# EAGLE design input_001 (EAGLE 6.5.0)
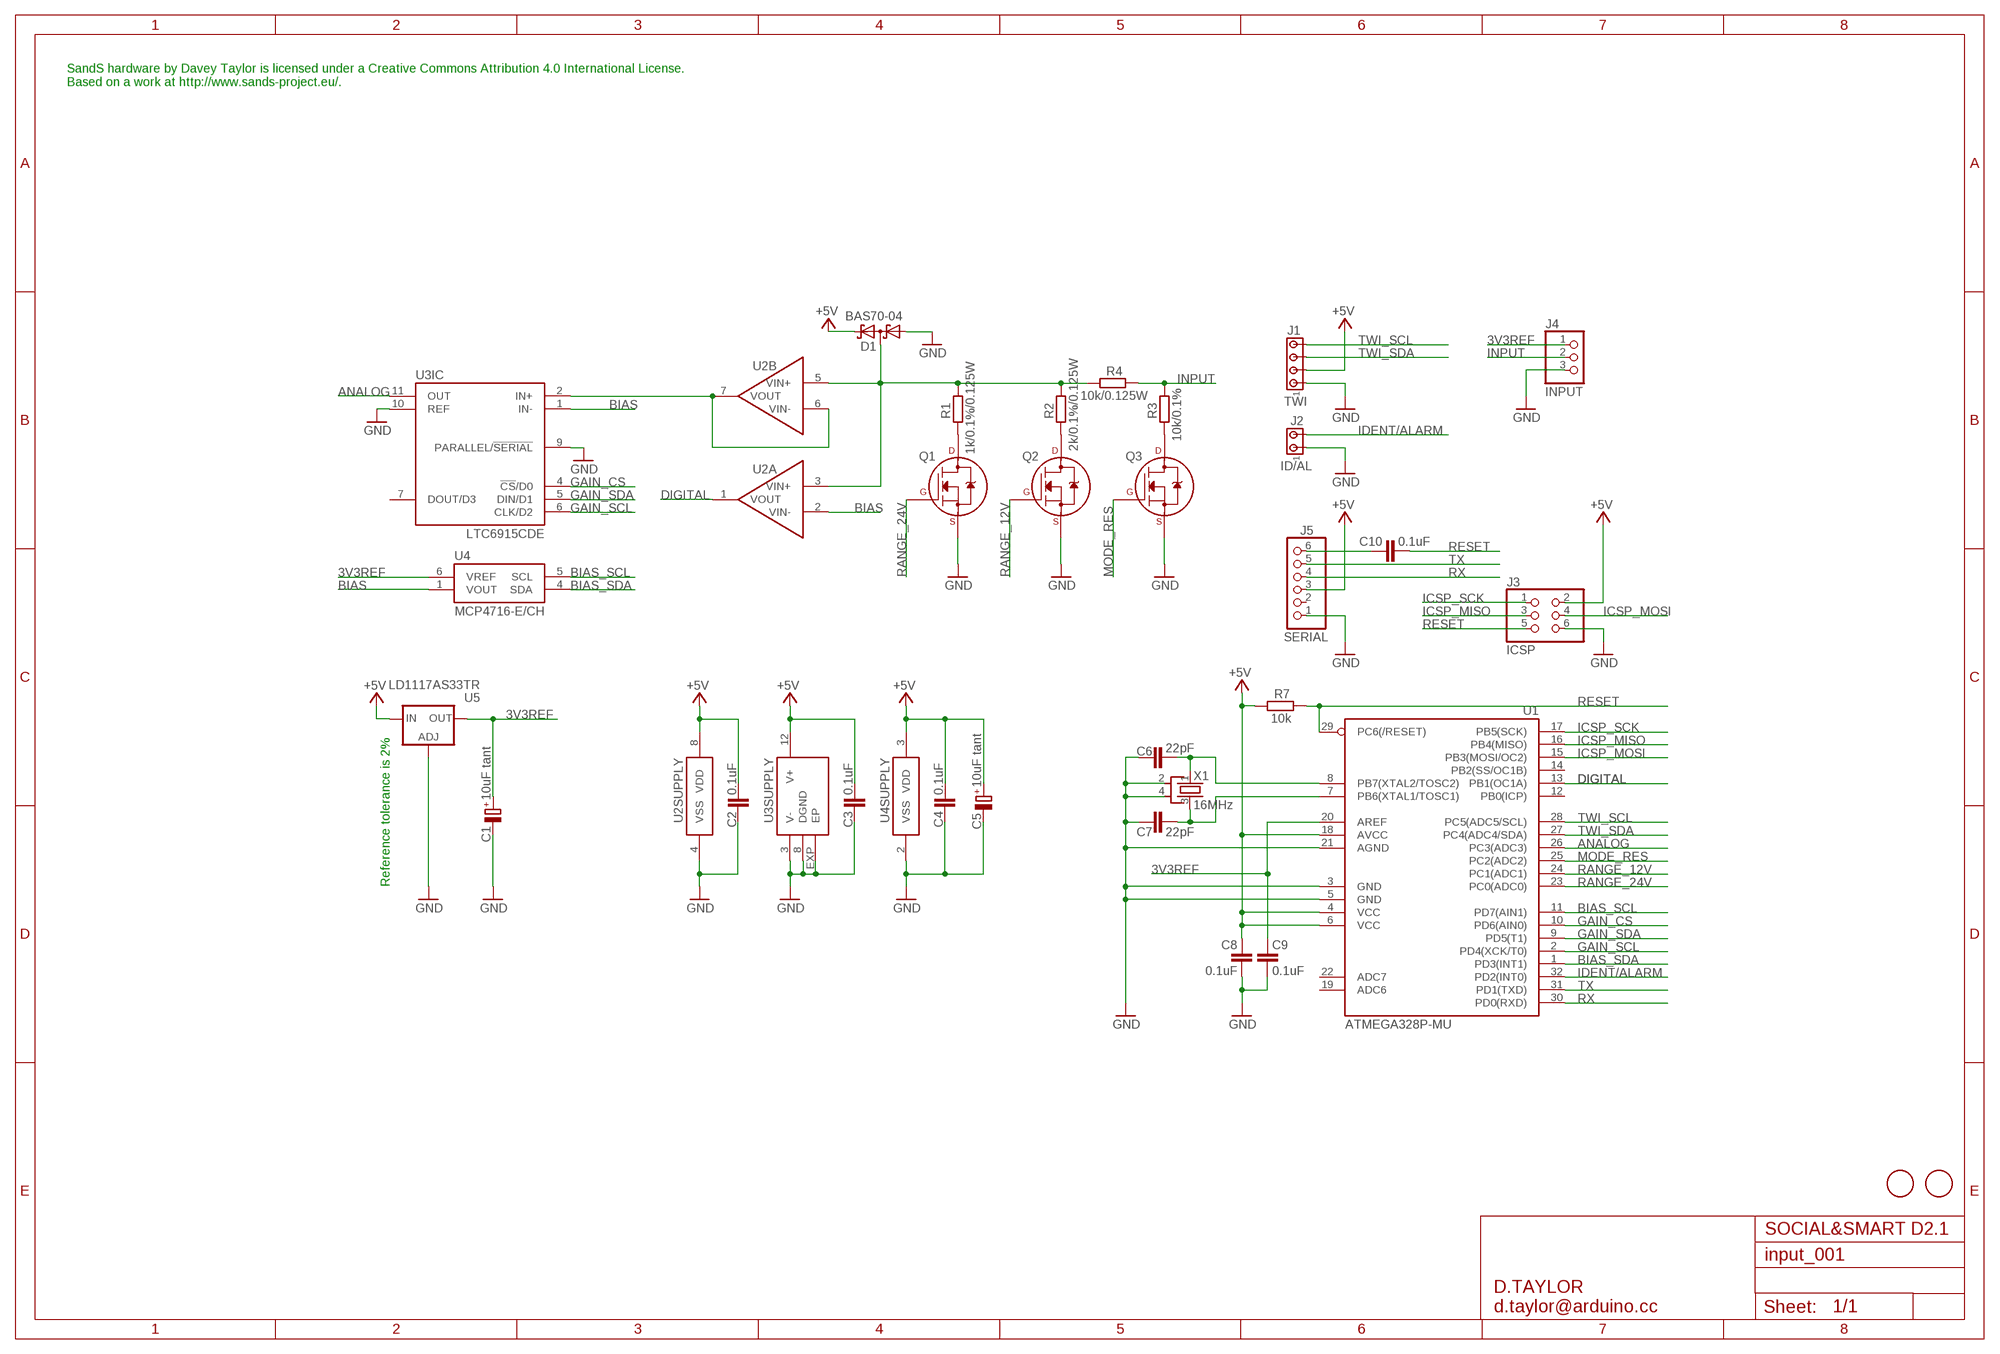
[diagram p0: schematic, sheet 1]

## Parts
C1  10uF tant  CPOL-EUSMCB  [SMC_B]
C2  0.1uF  C-EUC0603  [C0603]
C3  0.1uF  C-EUC0603  [C0603]
C4  0.1uF  C-EUC0603  [C0603]
C5  10uF tant  CPOL-EUSMCB  [SMC_B]
C6  22pF  C-EUC0603  [C0603]
C7  22pF  C-EUC0603  [C0603]
C8  0.1uF  C-EUC0603  [C0603]
C9  0.1uF  C-EUC0603  [C0603]
C10  0.1uF  C-EUC0603  [C0603]
D1  BAS70-04  [SOT23]
J1  TWI  MTA04-100  [10X04MTA]
J2  ID/AL  MTA02-100  [10X02MTA]
J3  ICSP  PINHD-2X3  [2X03]
J4  INPUT  MKDS_1,5/3-5,08  [MKDS1,5/3-5,08]
J5  SERIAL  PINHD-1X6  [1X06]
Q1  2N7002_SOT23  [SOT-23]
Q2  2N7002_SOT23  [SOT-23]
Q3  2N7002_SOT23  [SOT-23]
R1  1k/0.1%/0.125W  R-EU_R0603  [R0603]
R2  2k/0.1%/0.125W  R-EU_R0603  [R0603]
R3  10k/0.1%  R-EU_R0603  [R0603]
R4  10k/0.125W  R-EU_R0603  [R0603]
R7  10k  R-EU_R0603  [R0603]
U1  ATMEGA328P-MU  [MLF32-M1-A]
U2  MCP6402-E/SN  [SO8]
U3  LTC6915CDE  [DFN12]
U4  MCP4716-E/CH  [SOT-23-6]
U5  LD1117AS33TR  LD117AS33TR  [SOT223]
U$5  FIDUCIALMOUNT  [FIDUCIA-MOUNT]
U$6  FIDUCIALMOUNT  [FIDUCIA-MOUNT]
X1  16MHz  CRYSTAL-KX7  [XTAL-3.2-2.5]

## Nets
3V3REF: C1.+ C9.1 J4.1 U1.20(AREF) U4.6(VREF) U5.4(OUT)
+5V: C2.1 C3.1 C4.1 C5.+ C8.1 D1.2(C2) J1.2 J3.2 J5.3 R7.1 U1.4(VCC) U1.6(VCC) U1.18(AVCC) U2.8(SUPPLY:VDD) U3.12(SUPPLY:V+) U4.3(VDD) U5.3(IN)
ANALOG: U1.26(PC3(ADC3)) U3.11(IC:OUT)
BIAS: U2.2(A:VIN-) U3.1(IC:IN-) U4.1(VOUT)
BIAS_SCL: U1.11(PD7(AIN1)) U4.5(SCL)
BIAS_SDA: U1.1(PD3(INT1)) U4.4(SDA)
DIGITAL: U1.13(PB1(OC1A)) U2.1(A:VOUT)
GAIN_CS: U1.10(PD6(AIN0)) U3.4(IC:!CS!/D0)
GAIN_SCL: U1.2(PD4(XCK/T0)) U3.6(IC:CLK/D2)
GAIN_SDA: U1.9(PD5(T1)) U3.5(IC:DIN/D1)
GND: C1.- C2.2 C3.2 C4.2 C5.- C6.1 C7.1 C8.2 C9.2 D1.1(A1) J1.1 J2.1 J3.6 J4.3 J5.1 Q1.2(S) Q2.2(S) Q3.2(S) U1.3(GND) U1.5(GND) U1.21(AGND) U2.4(SUPPLY:VSS) U3.3(SUPPLY:V-) U3.8(SUPPLY:DGND) U3.9(IC:PARALLEL/!SERIAL) U3.10(IC:REF) U3.EXP(SUPPLY:EP) U4.2(VSS) U5.1(ADJ) X1.2(SH1) X1.4(SH2)
ICSP_MISO: J3.3 U1.16(PB4(MISO))
ICSP_MOSI: J3.4 U1.15(PB3(MOSI/OC2))
ICSP_SCK: J3.1 U1.17(PB5(SCK))
IDENT/ALARM: J2.2 U1.32(PD2(INT0))
INPUT: J4.2 R3.2 R4.2
MODE_RES: Q3.1(G) U1.25(PC2(ADC2))
N$1: Q1.3(D) R1.1
N$2: Q2.3(D) R2.1
N$3: Q3.3(D) R3.1
N$4: D1.3(C1A2) R1.2 R2.2 R4.1 U2.3(A:VIN+) U2.5(B:VIN+)
N$5: U2.6(B:VIN-) U2.7(B:VOUT) U3.2(IC:IN+)
N$6: C6.2 U1.8(PB7(XTAL2/TOSC2)) X1.1(X1)
N$7: C7.2 U1.7(PB6(XTAL1/TOSC1)) X1.3(X2)
N$9: C10.1 J5.6
RANGE_12V: Q2.1(G) U1.24(PC1(ADC1))
RANGE_24V: Q1.1(G) U1.23(PC0(ADC0))
RESET: C10.2 J3.5 R7.2 U1.29(PC6(/RESET))
RX: J5.4 U1.30(PD0(RXD))
TWI_SCL: J1.4 U1.28(PC5(ADC5/SCL))
TWI_SDA: J1.3 U1.27(PC4(ADC4/SDA))
TX: J5.5 U1.31(PD1(TXD))
Unconnected: J5.2 U1.12(PB0(ICP)) U1.14(PB2(SS/OC1B)) U1.19(ADC6) U1.22(ADC7) U3.7(IC:DOUT/D3)

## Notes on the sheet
- SandS hardware by Davey Taylor is licensed under a Creative Commons Attribution 4.0 International License.
  Based on a work at http://www.sands-project.eu/.
- Reference tolerance is 2%
- SOCIAL&SMART D2.1
- D.TAYLOR
  d.taylor@arduino.cc

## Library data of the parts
C1 C5 = rcl:CPOL-EU: POLARIZED CAPACITOR, European symbol
C2-C4 C6-C10 = rcl:C-EU: CAPACITOR, European symbol
D1 = diode:BAS70-04: Silicon Schottky Diodes General-purpose diode for high-speed switching
J1 = con-amp:MTA04-100: AMP connector
J2 = con-amp:MTA02-100: AMP connector
J3 = pinhead:PINHD-2X3: PIN HEADER
J4 = d_taylor:MKDS_1,5/3-5,08: MKDSN 1,5/ 3-5,08 Printklemme Nennstrom: 13,5 A Nennspannung: 250 V Rastermaß: 5,08 mm Polzahl: 3 Anschlussart: Schraubanschluss Montage: Löten Anschlussrichtung Leiter/Platine: 0 ° Artikelnummer: 1729131 Source: http://eshop.phoenixcontact.com .. 1729131.pdf; MPN: SMKDSN1,5/3-5,08; OC_FARNELL: 1792904; OC_NEWARK: 70R0299
J5 = pinhead:PINHD-1X6: PIN HEADER
Q1-Q3 = d_taylor:2N700*: 2N7000, 2N7002, NDS7002A N-channel enhancement mode MOSFET
R1-R4 R7 = rcl:R-EU_: RESISTOR, European symbol
U1 = d_taylor:ATMEGA*: MICROCONTROLLER 8 Kbytes FLASH 1 kbytes SRAM 512 bytes EEPROM USART 6-channel 10 bit ADC 2-channel 8 bit ADC Source: avr.lbr
U2 = d_taylor:MCP6402
U3 = d_taylor:LTC6915*DE
U4 = d_taylor:MCP47*6
U5 = v-reg:LD117A?*: Low drop fixed and adjustable positive voltage regulators 1 A Source: http://www.st.com/stonline/products/literature/ds/7194/ld1117axx.pdf
U$5 U$6 = SmartPrj:FIDUCIALMOUNT
X1 = d_taylor:CRYSTAL-KX7

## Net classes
1 PWR: width 0.406 mm, clearance 0.254 mm

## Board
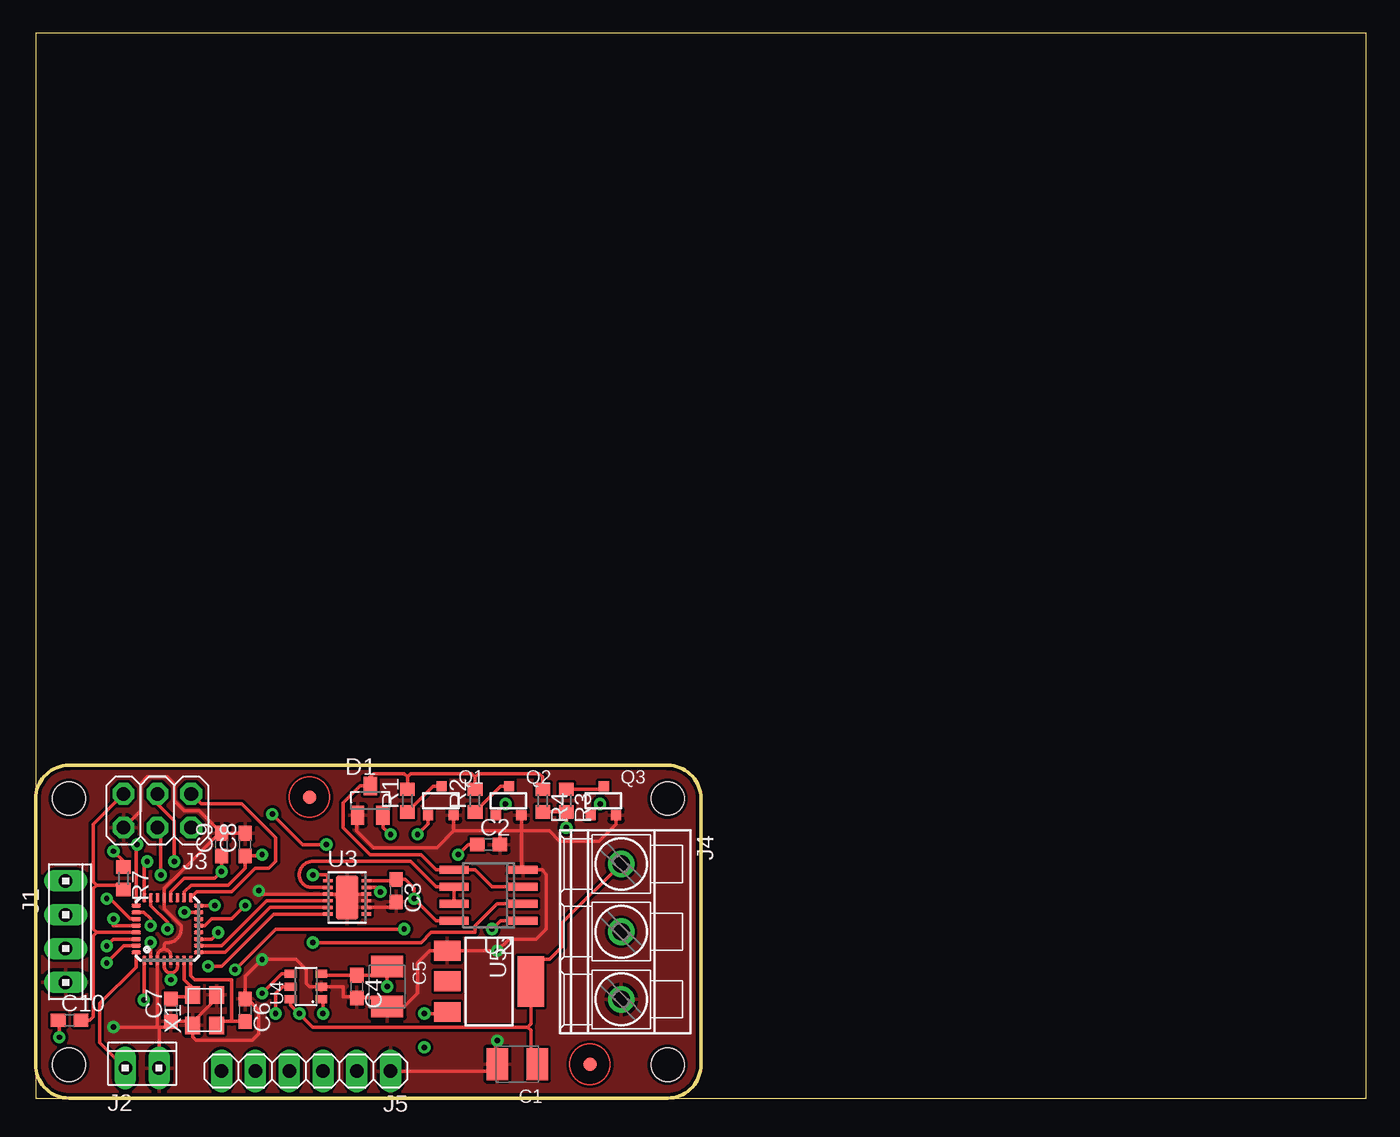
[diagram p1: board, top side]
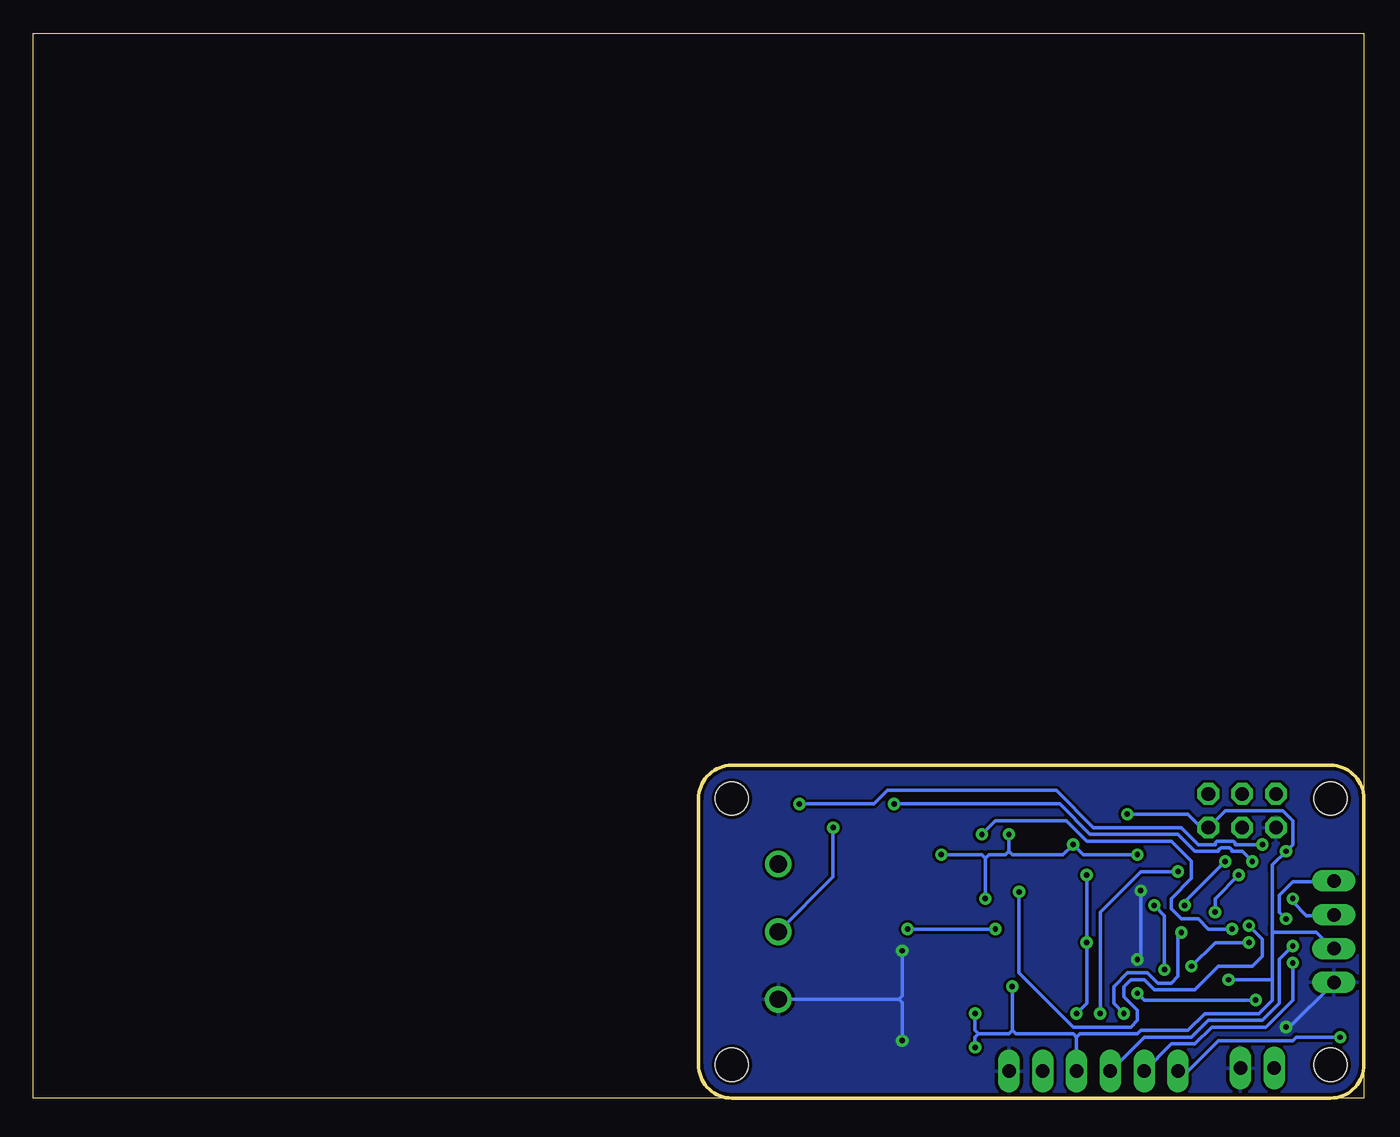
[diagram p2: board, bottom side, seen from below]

Size 100 x 80 mm. Coordinates in mm from the lower left corner, seen from the top.
Outline: 0,0 100,0 100,80 0,80 0,0
Outline: 2.5,0 47.5,0 arc90 50,2.5 50,22.5 arc90 47.5,25 2.5,25 arc90 0,22.5 0,2.5 arc90 2.5,0
Copper layers (1*16): Top 0.035mm / dielectric 1.5mm / Bottom 0.035mm
Design rules "smartprj-mini *": minimum track width 8mil, minimum drill 16mil, track to track 8mil, track to pad 8mil, pad to pad 0.200659375mm, via to via 8mil, smd to smd 4mil, copper to edge 10mil, drill to drill 8mil, minimum pad ring 12mil, minimum via ring 10mil, stop-mask expansion 2mil, vias tented up to drill 20mil, thermal gap 10mil
Holes 2.5 mm at 2.5,22.5 2.5,2.5 47.5,2.5 47.5,22.5

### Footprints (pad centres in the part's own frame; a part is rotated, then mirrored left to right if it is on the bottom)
SMC_B = smd 1.6 x 2.4: + -1.5,0; - 1.5,0
C0603 = smd 1.1 x 1: 1 -0.85,0; 2 0.85,0
SOT23 = smd 1 x 1.4: 1 -0.95,-1.1; 2 0.95,-1.1; 3 0,1.1
10X04MTA = drill 1.016 long: 1 3.81,0; 2 1.27,0; 3 -1.27,0; 4 -3.81,0
10X02MTA = drill 1.016 long: 1 1.27,0; 2 -1.27,0
2X03 = drill 1.016 octagon: 1 -2.54,-1.27; 2 -2.54,1.27; 3 0,-1.27; 4 0,1.27; 5 2.54,-1.27; 6 2.54,1.27
MKDS1,5/3-5,08 = drill 1.3 pad 2: 1 -5.08,0; 2 0,0; 3 5.08,0
1X06 = drill 1.016 long: 1 -6.35,0; 2 -3.81,0; 3 -1.27,0; 4 1.27,0; 5 3.81,0; 6 6.35,0
SOT-23 = smd 0.762 x 0.762: 1 -0.979,-1.101; 2 0.94,-1.101; 3 0.025,1.067
R0603 = smd 1 x 1.1: 1 -0.85,0; 2 0.85,0
MLF32-M1-A = smd 0.7 x 0.3: 1 -2.35,1.75; 2 -2.35,1.25; 3 -2.35,0.75; 4 -2.35,0.25; 5 -2.35,-0.25; 6 -2.35,-0.75; 7 -2.35,-1.25; 8 -2.35,-1.75; 17 2.35,-1.75; 18 2.35,-1.25; 19 2.35,-0.75; 20 2.35,-0.25; 21 2.35,0.25; 22 2.35,0.75; 23 2.35,1.25; 24 2.35,1.75 | smd 0.3 x 0.7: 9 -1.75,-2.35; 10 -1.25,-2.35; 11 -0.75,-2.35; 12 -0.25,-2.35; 13 0.25,-2.35; 14 0.75,-2.35; 15 1.25,-2.35; 16 1.75,-2.35; 25 1.75,2.35; 26 1.25,2.35; 27 0.75,2.35; 28 0.25,2.35; 29 -0.25,2.35; 30 -0.75,2.35; 31 -1.25,2.35; 32 -1.75,2.35
SO8 = smd 0.6 x 2.2: 1 -1.905,-2.6; 2 -0.635,-2.6; 3 0.635,-2.6; 4 1.905,-2.6; 5 1.905,2.6; 6 0.635,2.6; 7 -0.635,2.6; 8 -1.905,2.6
DFN12 = smd 0.25 x 0.7: 1 -1.25,-1.45; 2 -0.75,-1.45; 3 -0.25,-1.45; 4 0.25,-1.45; 5 0.75,-1.45; 6 1.25,-1.45; 7 1.25,1.45; 8 0.75,1.45; 9 0.25,1.45; 10 -0.25,1.45; 11 -0.75,1.45; 12 -1.25,1.45 | smd 3.3 x 1.7: EXP 0,0
SOT-23-6 = smd 0.6 x 0.9: 1 -0.95,-1.15; 2 0,-1.15; 3 0.95,-1.15; 4 0.95,1.15; 5 0,1.15; 6 -0.95,1.15
SOT223 = smd 1.5 x 2: 1 -2.3,-3.15; 2 0,-3.15; 3 2.3,-3.15 | smd 3.8 x 2: 4 0,3.15
FIDUCIA-MOUNT = smd 1.016 x 1.016: P$1 0,0
XTAL-3.2-2.5 = smd 1.3 x 1.1: 1 -1.15,-0.9; 2 1.15,-0.9; 3 1.15,0.9; 4 -1.15,0.9

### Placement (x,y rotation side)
C1  36.19,2.55 180 top
C2  34.04,19.05 0 top
C3  27.09,15.59 270 top
C4  24.13,8.38 270 top
C5  26.42,8.38 270 top
C6  15.75,6.6 270 top
C7  10.16,6.6 90 top
C8  15.75,19.05 90 top
C9  13.97,19.05 90 top
C10  2.54,5.84 0 top
D1  25.15,22.35 0 top
J1  2.25,12.5 270 top
J2  8,2.25 0 top
J3  9.14,21.59 180 top
J4  44,12.5 270 top
J5  20.32,2.03 180 top
Q1  30.48,22.35 0 top
Q2  35.56,22.35 0 top
Q3  42.67,22.35 0 top
R1  27.94,22.35 90 top
R2  33.02,22.35 90 top
R3  39.88,22.35 270 top
R4  38.1,22.35 270 top
R7  6.6,16.51 270 top
U1  9.91,12.7 90 top
U2  34.04,15.24 90 top
U3  23.4,15.08 270 top
U4  20.32,8.38 90 top
U5  34.07,8.77 270 top
U$5  20.57,22.61 0 top
U$6  41.66,2.54 0 top
X1  12.7,6.6 90 top

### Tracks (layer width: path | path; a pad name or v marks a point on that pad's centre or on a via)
3V3REF  (via drill 0.41)
  Top 0.254: C1.+ 37.22,3.02 37.22,5.08 36.97,5.33 | 19.17,7.37 U4.6 19.17,7.37 | U1.20 10.16,15.49 11.17,16.51 13.46,16.51 v13.97,17.02 C9.1 | J4.1 39.62,13.26 39.62,11.43 38.61,10.41 37.22,10.41 U5.4 37.22,5.59 36.97,5.33 | 19.17,7.37 19.17,6.99 v19.81,6.35 20.83,5.33 36.97,5.33
  Bottom 0.254: v19.81,6.35 19.81,13.97 16.76,17.02 v13.97,17.02
+5V  (via drill 0.41)
  Top 0.254: 11.18,15.32 U1.18 11.18,15.05 11.18,15.49 11.68,16 14.22,16 14.48,16 15.75,17.27 C8.1 | U3.12 26.95,16.33 C3.1 27.76,16.43 28.45,15.75 v28.45,14.99 30.1,13.34 U2.8 | 26.42,9.23 C4.1 21.47,9.23 U4.3 | 26.42,9.23 C5.+ v26.42,8.38 | 26.42,9.23 26.16,9.23 | D1.2 26.1,20.32 v26.67,19.81 | C2.1 32.51,19.05 v31.75,18.29 | C8.1 15.75,18.54 | R7.1 6.6,17.78 v5.84,18.54 | C8.1 16.93,18.2 v17.02,18.29 | v17.78,21.34 20.07,19.05 v21.84,19.05 | U1.4 9.66,9.9 arc90 10.16,9.4 | 10.16,9.4 arc90 10.66,9.89 U1.6 | 10.16,9.4 v10.16,8.89 | U5.3 30.81,6.35 v29.21,6.35
  Bottom 0.254: 29.21,4.57 28.96,4.83 | 28.96,4.83 26.67,4.83 26.42,5.08 | 26.42,5.08 26.16,4.83 21.84,4.83 21.59,4.57 | 21.59,4.57 21.34,4.83 17.02,4.83 16.76,5.08 13.21,5.08 11.94,6.35 7.87,6.35 7.37,6.86 6.86,7.37 6.86,8.89 | 29.21,4.57 v29.21,3.81 29.21,4.57 | 6.86,12.95 6.86,15.75 6.86,17.02 6.86,17.53 v5.84,18.54 5.33,19.05 5.33,20.83 6.1,21.59 10.41,21.59 J3.2 12.19,20.32 13.21,21.34 v17.78,21.34 | 6.86,12.95 6.86,12.45 | 6.86,12.45 3.56,12.45 2.25,11.18 J1.2 | v26.67,19.81 26.67,18.54 | 28.45,18.03 v28.45,14.99 | v31.75,18.29 28.7,18.29 28.45,18.03 | 26.67,18.54 26.42,18.29 22.61,18.29 v21.84,19.05 21.08,18.29 v17.02,18.29 | 6.86,12.45 6.86,12.95 | 6.86,12.95 6.86,8.89 | J5.3 21.59,4.57 | v10.16,8.89 6.86,8.89 | 26.67,18.54 26.92,18.29 28.19,18.29 28.45,18.03 | v26.42,8.38 26.42,5.08 | v29.21,6.35 29.21,5.08 28.96,4.83
ANALOG  (via drill 0.41)
  Top 0.254: U1.26 arc-90 7.58,13.97 8.13,13.97 8.64,13.46 v8.64,12.95 | U3.11 25.57,15.83 v25.91,15.49
  Bottom 0.254: v8.64,12.95 7.62,11.94 7.62,10.67 8.38,9.91 10.92,9.91 12.7,8.13 15.75,8.13 16.51,8.89 17.53,8.89 18.03,8.38 18.03,7.62 17.02,6.6 17.02,5.84 17.53,5.33 21.84,5.33 25.4,8.89 25.91,9.4 v25.91,15.49
BIAS  (via drill 0.41)
  Top 0.254: U4.1 21.47,7.37 21.59,7.37 v21.59,6.35 | v20.83,11.68 28.96,11.68 29.72,12.45 33.02,12.45 33.02,12.95 34.67,14.61 U2.2 | U3.1 21.95,16.76 v20.83,16.76
  Bottom 0.254: v20.83,16.76 v20.83,11.68 20.83,7.11 v21.59,6.35
BIAS_SCL  (via drill 0.41)
  Top 0.254: 12.26,11.94 U1.11 13.22,11.95 v13.72,12.45 | U4.5 18.54,8.38 18.03,7.87 v18.03,6.35
  Bottom 0.254: v13.72,12.45 13.97,12.19 13.97,9.14 14.48,8.64 15.49,8.64 16.26,9.4 17.78,9.4 18.8,8.38 18.8,7.11 v18.03,6.35
BIAS_SDA  (via drill 0.41)
  Top 0.254: U4.4 18.48,9.33 v17.02,7.87 | U1.1 8.16,7.39 v8.13,7.37
  Bottom 0.254: v8.13,7.37 16.51,7.37 v17.02,7.87
DIGITAL  (via drill 0.41)
  Top 0.254: U1.13 12.7,12.95 13.21,13.46 14.73,13.46 v15.75,14.48 | v14.99,9.65 18.03,12.7 27.18,12.7 v27.69,12.7 | U2.1 34.92,13.34 v34.29,12.7
  Bottom 0.254: v15.75,14.48 14.99,13.72 v14.99,9.65 | v34.29,12.7 v27.69,12.7
GAIN_CS
  Top 0.254: 12.26,11.43 U1.10 13.97,11.45 17.35,14.83 U3.4
GAIN_SCL  (via drill 0.41)
  Top 0.254: U1.2 8.66,11.94 v8.64,11.68 | v12.95,9.91 13.97,9.91 17.89,13.83 U3.6
  Bottom 0.254: v8.64,11.68 11.18,11.68 v12.95,9.91
GAIN_SDA
  Top 0.254: 12.19,10.92 12.19,10.95 U1.9 14.25,10.95 17.63,14.33 U3.5
GND  (via drill 0.41)
  Top 0.254: 13.85,7.62 X1.2 13.6,7.5 12.7,6.6 11.8,5.7 X1.4 | 12.05,5.75 X1.4 | C3.2 26.94,14.33 U3.8 U3.9 U3.10 23.4,15.33 | C9.2 C8.2 C9.2 | C4.2 24.64,7.53 | 24.64,7.53 26.42,7.53 C5.- 27.71,6.88 28.7,7.87 28.7,10.16 29.61,11.07 U5.1 34.29,11.07 | 24.64,7.53 24.64,7.62 23.11,7.62 23.11,8.38 U4.2 20.57,8.38 20.32,8.64 20.32,9.65 19.56,10.41 v17.02,10.41 15.75,9.14 C6.1 15.91,7.45 16.76,6.6 16.76,4.83 16.26,4.35 12.05,4.35 11.8,4.6 X1.4 | 10.16,10.16 U1.5 10.16,10.68 arc90 9.66,11.18 | 9.14,10.35 U1.3 9.14,10.35 | 9.65,11.18 9.66,11.18 | 9.66,11.18 9.66,11.43 arc-90 9.91,11.68 arc90 10.92,12.7 10.92,12.95 9.65,14.22 U1.21 9.65,15.75 10.92,17.02 13.8,19.9 C9.2 | v34.69,11.07 34.29,11.07 | Q1.2 31.42,20.07 | D1.1 24.13,21.25 24.13,20.07 25.4,18.8 29.21,18.8 30.15,18.8 31.42,20.07 | 31.42,20.07 34.8,20.07 | 34.8,20.07 36.5,20.07 | 36.5,20.07 Q2.2 | 36.5,20.07 38.61,20.07 39.37,19.3 42.34,19.3 43.61,20.57 Q3.2 | v34.69,11.07 34.29,11.07 | 9.14,10.35 9.14,6.6 9.14,5.33 | J2.1 9.27,4.06 9.27,4.35 9.27,5.33 9.14,5.33 | J5.1 34.69,2.03 C1.- 34.54,2.55 34.54,4.17 v34.69,4.32 | 23.4,15.33 U3.3 17.02,15.33 v16.76,15.58 | 23.4,15.33 U3.EXP 23.4,15.33 | X1.4 11.8,5.75 C7.1 9.74,5.33 9.14,5.33 | v5.84,5.33 6.35,5.33 8.38,5.33 9.14,5.33 | 9.14,10.35 9.14,10.66 arc-90 9.66,11.18 | J3.6 7.87,21.59 7.87,23.62 8.38,24.13 9.91,24.13 10.41,23.62 10.41,22.35 11.18,21.59 12.28,21.59 C9.2 | 36.5,20.07 36.5,17.28 U2.4 38.1,17.14 38.35,16.76 38.35,12.7 37.59,11.94 35.56,11.94 v34.69,11.07 | C2.2 34.89,19.98 34.8,20.07
  Bottom 0.254: v34.69,4.32 34.69,5.33 34.69,7.17 34.95,7.42 | J4.3 34.95,7.42 | J1.1 2.25,8.64 5.59,5.33 v5.84,5.33 | v17.02,10.41 16.76,10.76 v16.76,15.58 | v34.69,11.07 34.69,7.67 34.95,7.42
  pour Top: 0.5,22.5 arc-90 2.5,24.5 47.5,24.5 arc-90 49.5,22.5 49.5,2.5 arc-90 47.5,0.5 2.5,0.5 arc-90 0.5,2.5
  pour Bottom: 0.5,22.5 arc-90 2.5,24.5 47.5,24.5 arc-90 49.5,22.5 49.5,2.5 arc-90 47.5,0.5 2.5,0.5 arc-90 0.5,2.5
ICSP_MISO  (via drill 0.41)
  Top 0.254: J3.3 9.14,22.1 10.41,20.83 10.41,19.56 v10.41,17.78 | v13.46,14.48 13.72,14.45 U1.16
  Bottom 0.254: v10.41,17.78 13.46,14.73 v13.46,14.48
ICSP_MOSI  (via drill 0.41)
  Top 0.254: J3.4 9.4,20.07 v9.4,16.76 | U1.15 11.2,13.95 v11.18,13.97
  Bottom 0.254: v9.4,16.76 11.18,14.99 v11.18,13.97
ICSP_SCK
  Top 0.254: J3.1 12.45,22.1 15.49,22.1 18.03,19.56 18.03,17.78 17.53,17.27 16.51,17.27 14.73,15.49 12.1,15.49 U1.17
IDENT/ALARM
  Top 0.254: J2.2 4.83,4.16 4.83,7.11 7.56,9.84 U1.32
INPUT  (via drill 0.41)
  Top 0.254: R4.2 R3.2 v39.88,20.32
  Bottom 0.254: J4.2 39.88,16.62 v39.88,20.32
MODE_RES  (via drill 0.41)
  Top 0.254: U1.25 7.56,18.86 v7.62,19.05 | Q3.1 41.69,21.37 v42.42,22.1
  Bottom 0.254: v7.62,19.05 8.13,19.05 9.65,19.05 arc-90 9.91,19.3 10.41,19.3 10.92,19.3 arc-90 11.18,19.05 12.45,19.05 13.72,20.32 20.32,20.32 23.11,23.11 35.81,23.11 36.83,22.1 v42.42,22.1
N$1
  Top 0.254: Q1.3 29.86,23.42 R1.1
N$2
  Top 0.254: Q2.3 34.94,23.42 R2.1
N$3
  Top 0.254: R3.1 42.48,23.2 Q3.3
N$4
  Top 0.254: 24.77,18.67 23.11,20.32 23.11,22.18 24.38,23.45 D1.3 25.15,24.13 25.4,24.38 27.69,24.38 27.94,24.13 | 24.77,18.67 25.15,18.29 | 36.83,15.75 36.64,15.75 U2.3 34.29,15.88 33.02,17.14 U2.5 30.73,17.14 30.1,17.14 28.96,18.29 25.15,18.29 | R1.2 27.94,24.13 | 27.94,24.13 28.19,24.38 32.77,24.38 33.02,24.13 | 33.02,24.13 R2.2 33.02,24.13 | 33.02,24.13 33.27,24.38 37.85,24.38 38.1,24.13 R4.1 | 25.15,18.29 24.77,18.67
N$5
  Top 0.254: U2.7 U2.6 30.1,15.88 28.19,17.78 20.83,17.78 arc90 19.81,16.76 arc90 20.75,15.83 U3.2
N$6
  Top 0.254: C6.2 14.73,5.75 | 14.73,5.75 14.73,8.89 11.94,8.89 11.68,9.14 11.66,9.17 U1.8 | 14.73,5.75 13.9,5.75 X1.1
N$7
  Top 0.254: C7.2 10.16,7.62 12.05,7.62 X1.3 11.94,7.75 11.94,8.13 11.16,8.89 U1.7
N$9  (via drill 0.41)
  Top 0.254: v1.78,4.57 1.78,5.84 C10.1
  Bottom 0.254: J5.6 13.21,2.03 10.92,4.32 5.33,4.32 5.08,4.57 v1.78,4.57
RANGE_12V  (via drill 0.41)
  Top 0.254: U1.24 8.16,17.55 v8.38,17.78 | Q2.1 34.58,21.37 v35.31,22.1
  Bottom 0.254: v8.38,17.78 9.14,18.54 9.91,18.54 arc-90 10.16,18.8 10.41,18.8 10.67,18.8 arc-90 10.92,18.54 12.7,18.54 13.97,19.81 20.57,19.81 22.86,22.1 v35.31,22.1
RANGE_24V  (via drill 0.41)
  Top 0.254: U1.23 8.66,14.46 9.91,13.21 v9.91,12.7 | Q1.1 29.5,20.61 v28.7,19.81
  Bottom 0.254: v9.91,12.7 11.68,12.7 12.45,13.46 13.72,13.46 14.48,14.22 14.48,14.99 12.95,16.51 12.95,17.78 14.48,19.3 20.83,19.3 22.35,20.83 25.65,20.83 27.69,20.83 v28.7,19.81
RESET
  Top 0.254: U1.29 5.84,12.45 4.57,12.45 | 4.57,12.45 4.32,12.7 4.32,15.75 4.57,16 | 4.57,16 4.32,16.26 4.32,20.57 J3.5 | C10.2 4.06,5.84 4.32,6.1 4.32,12.19 4.57,12.45 | R7.2 6.6,16 4.57,16
RX  (via drill 0.41)
  Top 0.254: U1.30 7.56,11.94 5.84,11.94 v5.33,11.43
  Bottom 0.254: v5.33,11.43 6.35,10.41 6.35,7.11 6.86,6.6 7.62,5.84 11.68,5.84 12.95,4.57 16.51,4.57 J5.4
TWI_SCL  (via drill 0.41)
  Top 0.254: U1.28 5.84,12.95 v5.84,13.46
  Bottom 0.254: v5.84,13.46 6.35,13.97 6.35,15.24 5.33,16.26 2.29,16.26 2.29,16.31 J1.4
TWI_SDA  (via drill 0.41)
  Top 0.254: v5.33,14.99 5.59,14.99 7.11,13.46 7.56,13.46 U1.27
  Bottom 0.254: J1.3 2.25,13.72 4.32,13.72 5.33,14.73 v5.33,14.99
TX  (via drill 0.41)
  Top 0.254: U1.31 6.6,11.45 v5.33,10.16
  Bottom 0.254: v5.33,10.16 5.33,7.37 7.37,5.33 11.43,5.33 12.7,4.06 14.48,4.06 J5.5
